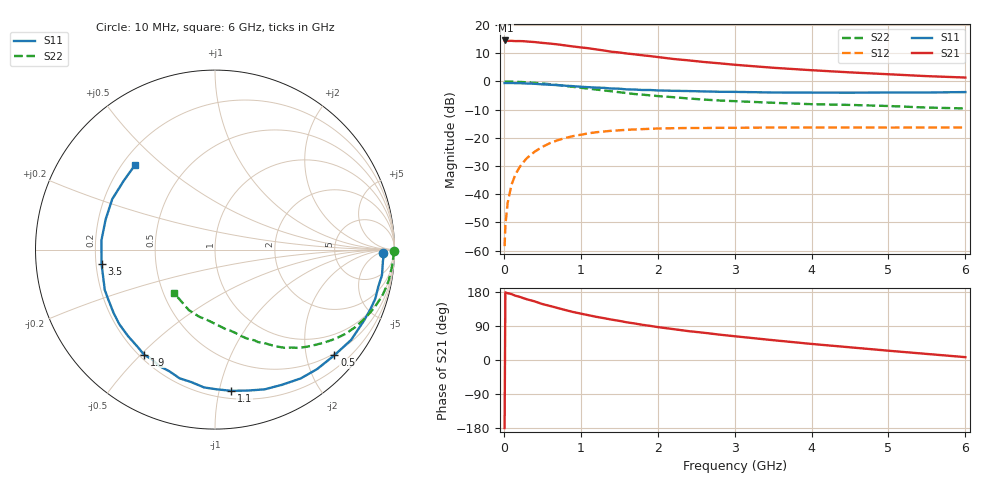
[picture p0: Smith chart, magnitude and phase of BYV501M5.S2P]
! SIEMENS Small Signal Semiconductors
! BFY420
! Si NPN RF SIEGET Grounded Emitter Transistor in MICRO-X
! VCE = 0.5 V  IC = 1.5 mA
! Common Emitter S-Parameters:  October  1996
# GHz  S  MA  R  50
!  f  S11  S21  S12  S22
! GHz  MAG  ANG  MAG  ANG  MAG  ANG  MAG  ANG
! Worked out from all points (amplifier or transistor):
!   36 points, 10 MHz to 6 GHz, reference 50 ohm
!   highest |S21| = 14.5 dB at 20 MHz (marker M1)
!   |S21| within 3 dB of that: start of sweep to 1.158 GHz
!   unconditionally stable (mu >= 1): 4.188 GHz to end of sweep
!   at 250 MHz: K = 0.06, MSG = 21.5 dB, |S12| = -28.7 dB
!   at 1.4 GHz: K = 0.30, MSG = 14.0 dB, |S12| = -17.5 dB
!   at 6 GHz: K = 1.31, MAG = 5.5 dB, |S12| = -16.3 dB
!   S11 on the Smith chart (normalised r, x): 10 MHz: 29, -9; 500 MHz: 0.46, -2.57; 1.1 GHz: 0.26, -1.09; 1.9 GHz: 0.22, -0.51; 3.5 GHz: 0.22, -0.06; 6 GHz: 0.25, +0.41
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0.01  0.9383 -1.1  5.327 -179.5  0.0012 88.7  0.9949 -0.5
0.02  0.9401 -2.0  5.338 178.4  0.0028 95.2  0.996 -1.0
0.05  0.9378 -4.2  5.24 176.2  0.0071 89.4  0.9943 -2.5
0.1  0.9412 -8.7  5.255 173.9  0.0148 86.2  0.9911 -5.1
0.15  0.9329 -12.8  5.198 169.6  0.0224 81.4  0.9863 -7.7
0.25  0.9272 -21.1  5.185 163.5  0.0366 76.2  0.9749 -12.7
0.4  0.9104 -33.5  5.001 154.7  0.0568 69.3  0.9457 -19.9
0.5  0.8883 -41.5  4.834 147.7  0.0692 64.2  0.9207 -24.4
0.7  0.8619 -56.4  4.544 137.2  0.0908 55.4  0.8648 -32.9
0.8  0.8405 -63.7  4.353 131.8  0.0995 50.9  0.8332 -36.7
0.9  0.8261 -70.5  4.173 126.7  0.1075 47.0  0.8025 -40.0
1.1  0.7922 -83.4  3.884 118.2  0.1202 40.3  0.7456 -46.5
1.4  0.7497 -100.2  3.366 106.6  0.1334 31.3  0.6705 -54.7
1.6  0.7239 -110.6  3.13 99.4  0.1389 26.7  0.6218 -59.1
1.9  0.7063 -124.1  2.822 90.1  0.1446 20.6  0.5678 -65.1
2.2  0.6832 -135.2  2.511 81.6  0.1484 15.5  0.527 -70.2
2.4  0.676 -142.1  2.368 76.2  0.1496 12.9  0.4996 -73.6
2.8  0.6567 -154.5  2.101 67.0  0.1507 8.3  0.4599 -79.2
3.5  0.6371 -172.9  1.751 52.3  0.1527 2.5  0.419 -88.4
4.5  0.632 164.5  1.45 33.5  0.1528 -4.2  0.3838 -103.5
5.5  0.6368 143.0  1.243 16.0  0.1523 -8.0  0.3445 -122.9
6  0.6489 133.4  1.174 7.5  0.1531 -9.1  0.3325 -134.0
